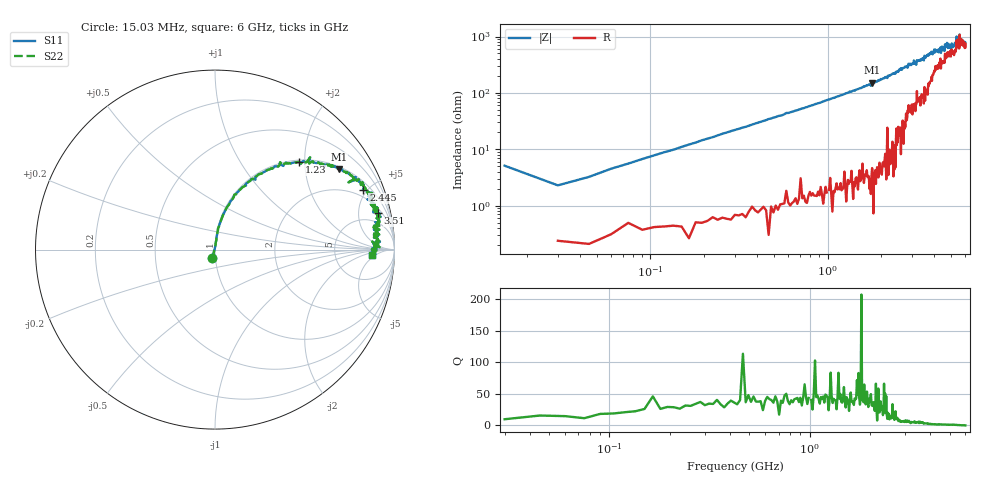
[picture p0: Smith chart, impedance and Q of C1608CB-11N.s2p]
!	Network	Analyzer	HP8753E.07.74:	Oct	30	2002	Serial	No.	JP38451487
!	Hewlett-Packard
!	28	Aug	2009	7:53:39
!	Frequency	S11	S21	S12	S22
#	HZ	S	RI	R	50
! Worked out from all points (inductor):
!   400 points, 15.03 MHz to 6 GHz, reference 50 ohm
!   read as one part in series: L = 11.8 nH near 45.03 MHz
!   highest Q = 48.1 at 1.785 GHz (marker M1), where L = 13.5 nH
!   self-resonance near 5.621 GHz
!   S11 on the Smith chart (normalised r, x): 15.03 MHz: 0.97, -0.10; 1.23 GHz: 1.04, +1.88; 2.445 GHz: 1.47, +4.74; 3.51 GHz: 2.76, +8.17; 6 GHz: 14, -3
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1.502992e7  -0.0152 -0.0491  1.02 0.0491  1.02 0.0491  -0.0152 -0.0491
3.002985e7  0.0028 0.0227  0.997 -0.0227  0.997 -0.0227  0.0028 0.0227
6.00297e7  0.00525 0.0448  0.995 -0.0448  0.995 -0.0448  0.00525 0.0448
1.050295e8  0.0103 0.077  0.99 -0.077  0.99 -0.077  0.0103 0.077
2.850286e8  0.0474 0.199  0.953 -0.199  0.953 -0.199  0.0474 0.199
5.850271e8  0.173 0.358  0.827 -0.358  0.827 -0.358  0.173 0.358
1.020025e9  0.372 0.471  0.628 -0.471  0.628 -0.471  0.372 0.471
1.230024e9  0.47 0.488  0.53 -0.488  0.53 -0.488  0.47 0.488
1.785021e9  0.691 0.447  0.309 -0.447  0.309 -0.447  0.691 0.447
2.01002e9  0.746 0.424  0.254 -0.424  0.254 -0.424  0.746 0.424
2.445018e9  0.827 0.332  0.173 -0.332  0.173 -0.332  0.827 0.332
3.015015e9  0.889 0.257  0.111 -0.257  0.111 -0.257  0.889 0.257
3.510012e9  0.907 0.202  0.0932 -0.202  0.0932 -0.202  0.907 0.202
4.00501e9  0.915 0.132  0.0849 -0.132  0.0849 -0.132  0.915 0.132
5.010005e9  0.892 0.0768  0.108 -0.0768  0.108 -0.0768  0.892 0.0768
5.295004e9  0.9 0.0747  0.1 -0.0747  0.1 -0.0747  0.9 0.0747
5.355003e9  0.919 0.0434  0.0811 -0.0434  0.0811 -0.0434  0.919 0.0434
5.535002e9  0.876 0.0448  0.124 -0.0448  0.124 -0.0448  0.876 0.0448
5.565002e9  0.917 0.0136  0.0833 -0.0136  0.0833 -0.0136  0.917 0.0136
5.595002e9  0.882 0.0345  0.118 -0.0345  0.118 -0.0345  0.882 0.0345
5.685002e9  0.901 0.0116  0.0988 -0.0116  0.0988 -0.0116  0.901 0.0116
6e9  0.872 -0.0278  0.128 0.0278  0.128 0.0278  0.872 -0.0278
